(* Logix 5000 AddOnInstructionDefinition export RTA_435NBX_490NBX_Heartbeat; software revision 20.01 *)

ADD_ON_INSTRUCTION RTA_435NBX_490NBX_Heartbeat   (* revision 1.0, vendor Real Time Automation, Inc. *)
// RTA's 435NBX / 490NBX Heartbeat Handshaking
VAR_IN_OUT
   DataIn : INT; {required}
   DataOut : INT; {required}
END_VAR
VAR
   Previous_Value : INT; {access None}
   Number_of_Times_Inactive : INT; {access None}
END_VAR

ROUTINE Logic   (* ladder *)
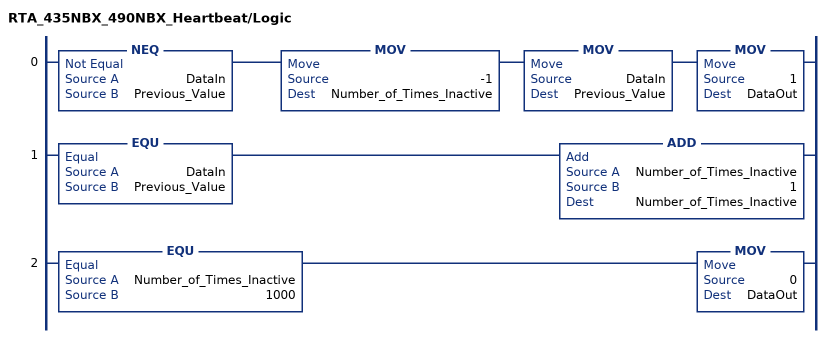
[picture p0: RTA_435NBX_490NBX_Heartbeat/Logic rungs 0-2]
   0: NEQ(DataIn,Previous_Value)MOV(-1,Number_of_Times_Inactive)MOV(DataIn,Previous_Value)MOV(1,DataOut);
   1: EQU(DataIn,Previous_Value)ADD(Number_of_Times_Inactive,1,Number_of_Times_Inactive);
   2: EQU(Number_of_Times_Inactive,1000)MOV(0,DataOut);
END_ROUTINE
END_ADD_ON_INSTRUCTION
